DATA_BLOCK DB 20
NAME : DB_LED
VERSION : 0.1


  STRUCT
   LED_0_0 : BOOL ;
   LED_0_1 : BOOL ;
   LED_0_2 : BOOL ;
   LED_0_3 : BOOL ;
   LED_0_4 : BOOL ;
   LED_0_5 : BOOL ;
   LED_0_6 : BOOL ;
   LED_0_7 : BOOL ;
   LED_1_0 : BOOL ;
   LED_1_1 : BOOL ;
   LED_1_2 : BOOL ;
   LED_1_3 : BOOL ;
   LED_1_4 : BOOL ;
   LED_1_5 : BOOL ;
   LED_1_6 : BOOL ;
   LED_1_7 : BOOL ;
   LED_2_0 : BOOL ;
   LED_2_1 : BOOL ;
   LED_2_2 : BOOL ;
   LED_2_3 : BOOL ;
   LED_2_4 : BOOL ;
   LED_2_5 : BOOL ;
   LED_2_6 : BOOL ;
   LED_2_7 : BOOL ;
   LED_3_0 : BOOL ;
   LED_3_1 : BOOL ;
   LED_3_2 : BOOL ;
   LED_3_3 : BOOL ;
   LED_3_4 : BOOL ;
   LED_3_5 : BOOL ;
   LED_3_6 : BOOL ;
   LED_3_7 : BOOL ;
   LED_4_0 : BOOL ;
   LED_4_1 : BOOL ;
   LED_4_2 : BOOL ;
   LED_4_3 : BOOL ;
   LED_4_4 : BOOL ;
   LED_4_5 : BOOL ;
   LED_4_6 : BOOL ;
   LED_4_7 : BOOL ;
   LED_5_0 : BOOL ;
   LED_5_1 : BOOL ;
   LED_5_2 : BOOL ;
   LED_5_3 : BOOL ;
   LED_5_4 : BOOL ;
   LED_5_5 : BOOL ;
   LED_5_6 : BOOL ;
   LED_5_7 : BOOL ;
   LED_6_0 : BOOL ;
   LED_6_1 : BOOL ;
   LED_6_2 : BOOL ;
   LED_6_3 : BOOL ;
   LED_6_4 : BOOL ;
   LED_6_5 : BOOL ;
   LED_6_6 : BOOL ;
   LED_6_7 : BOOL ;
   LED_7_0 : BOOL ;
   LED_7_1 : BOOL ;
   LED_7_2 : BOOL ;
   LED_7_3 : BOOL ;
   LED_7_4 : BOOL ;
   LED_7_5 : BOOL ;
   LED_7_6 : BOOL ;
   LED_7_7 : BOOL ;
   LED_8_0 : BOOL ;
   LED_8_1 : BOOL ;
   LED_8_2 : BOOL ;
   LED_8_3 : BOOL ;
   LED_8_4 : BOOL ;
   LED_8_5 : BOOL ;
   LED_8_6 : BOOL ;
   LED_8_7 : BOOL ;
   LED_9_0 : BOOL ;
   LED_9_1 : BOOL ;
   LED_9_2 : BOOL ;
   LED_9_3 : BOOL ;
   LED_9_4 : BOOL ;
   LED_9_5 : BOOL ;
   LED_9_6 : BOOL ;
   LED_9_7 : BOOL ;
   LED_10_0 : BOOL ;
   LED_10_1 : BOOL ;
   LED_10_2 : BOOL ;
   LED_10_3 : BOOL ;
   LED_10_4 : BOOL ;
   LED_10_5 : BOOL ;
   LED_10_6 : BOOL ;
   LED_10_7 : BOOL ;
   LED_11_0 : BOOL ;
   LED_11_1 : BOOL ;
   LED_11_2 : BOOL ;
   LED_11_3 : BOOL ;
   LED_11_4 : BOOL ;
   LED_11_5 : BOOL ;
   LED_11_6 : BOOL ;
   LED_11_7 : BOOL ;
   LED_12_0 : BOOL ;
   LED_12_1 : BOOL ;
   LED_12_2 : BOOL ;
   LED_12_3 : BOOL ;
   LED_12_4 : BOOL ;
   LED_12_5 : BOOL ;
   LED_12_6 : BOOL ;
   LED_12_7 : BOOL ;
   LED_13_0 : BOOL ;
   LED_13_1 : BOOL ;
   LED_13_2 : BOOL ;
   LED_13_3 : BOOL ;
   LED_13_4 : BOOL ;
   LED_13_5 : BOOL ;
   LED_13_6 : BOOL ;
   LED_13_7 : BOOL ;
   LED_14_0 : BOOL ;
   LED_14_1 : BOOL ;
   LED_14_2 : BOOL ;
   LED_14_3 : BOOL ;
   LED_14_4 : BOOL ;
   LED_14_5 : BOOL ;
   LED_14_6 : BOOL ;
   LED_14_7 : BOOL ;
   LED_15_0 : BOOL ;
   LED_15_1 : BOOL ;
   LED_15_2 : BOOL ;
   LED_15_3 : BOOL ;
   LED_15_4 : BOOL ;
   LED_15_5 : BOOL ;
   LED_15_6 : BOOL ;
   LED_15_7 : BOOL ;
   LED_16_0 : BOOL ;
   LED_16_1 : BOOL ;
   LED_16_2 : BOOL ;
   LED_16_3 : BOOL ;
   LED_16_4 : BOOL ;
   LED_16_5 : BOOL ;
   LED_16_6 : BOOL ;
   LED_16_7 : BOOL ;
   LED_17_0 : BOOL ;
   LED_17_1 : BOOL ;
   LED_17_2 : BOOL ;
   LED_17_3 : BOOL ;
   LED_17_4 : BOOL ;
   LED_17_5 : BOOL ;
   LED_17_6 : BOOL ;
   LED_17_7 : BOOL ;
   LED_18_0 : BOOL ;
   LED_18_1 : BOOL ;
   LED_18_2 : BOOL ;
   LED_18_3 : BOOL ;
   LED_18_4 : BOOL ;
   LED_18_5 : BOOL ;
   LED_18_6 : BOOL ;
   LED_18_7 : BOOL ;
   LED_19_0 : BOOL ;
   LED_19_1 : BOOL ;
   LED_19_2 : BOOL ;
   LED_19_3 : BOOL ;
   LED_19_4 : BOOL ;
   LED_19_5 : BOOL ;
   LED_19_6 : BOOL ;
   LED_19_7 : BOOL ;
   LED_20_0 : BOOL ;
   LED_20_1 : BOOL ;
   LED_20_2 : BOOL ;
   LED_20_3 : BOOL ;
   LED_20_4 : BOOL ;
   LED_20_5 : BOOL ;
   LED_20_6 : BOOL ;
   LED_20_7 : BOOL ;
   LED_21_0 : BOOL ;
   LED_21_1 : BOOL ;
   LED_21_2 : BOOL ;
   LED_21_3 : BOOL ;
   LED_21_4 : BOOL ;
   LED_21_5 : BOOL ;
   LED_21_6 : BOOL ;
   LED_21_7 : BOOL ;
  END_STRUCT ;
BEGIN
   LED_0_0 := FALSE;
   LED_0_1 := FALSE;
   LED_0_2 := FALSE;
   LED_0_3 := FALSE;
   LED_0_4 := FALSE;
   LED_0_5 := FALSE;
   LED_0_6 := FALSE;
   LED_0_7 := FALSE;
   LED_1_0 := FALSE;
   LED_1_1 := FALSE;
   LED_1_2 := FALSE;
   LED_1_3 := FALSE;
   LED_1_4 := FALSE;
   LED_1_5 := FALSE;
   LED_1_6 := FALSE;
   LED_1_7 := FALSE;
   LED_2_0 := FALSE;
   LED_2_1 := FALSE;
   LED_2_2 := FALSE;
   LED_2_3 := FALSE;
   LED_2_4 := FALSE;
   LED_2_5 := FALSE;
   LED_2_6 := FALSE;
   LED_2_7 := FALSE;
   LED_3_0 := FALSE;
   LED_3_1 := FALSE;
   LED_3_2 := FALSE;
   LED_3_3 := FALSE;
   LED_3_4 := FALSE;
   LED_3_5 := FALSE;
   LED_3_6 := FALSE;
   LED_3_7 := FALSE;
   LED_4_0 := FALSE;
   LED_4_1 := FALSE;
   LED_4_2 := FALSE;
   LED_4_3 := FALSE;
   LED_4_4 := FALSE;
   LED_4_5 := FALSE;
   LED_4_6 := FALSE;
   LED_4_7 := FALSE;
   LED_5_0 := FALSE;
   LED_5_1 := FALSE;
   LED_5_2 := FALSE;
   LED_5_3 := FALSE;
   LED_5_4 := FALSE;
   LED_5_5 := FALSE;
   LED_5_6 := FALSE;
   LED_5_7 := FALSE;
   LED_6_0 := FALSE;
   LED_6_1 := FALSE;
   LED_6_2 := FALSE;
   LED_6_3 := FALSE;
   LED_6_4 := FALSE;
   LED_6_5 := FALSE;
   LED_6_6 := FALSE;
   LED_6_7 := FALSE;
   LED_7_0 := FALSE;
   LED_7_1 := FALSE;
   LED_7_2 := FALSE;
   LED_7_3 := FALSE;
   LED_7_4 := FALSE;
   LED_7_5 := FALSE;
   LED_7_6 := FALSE;
   LED_7_7 := FALSE;
   LED_8_0 := FALSE;
   LED_8_1 := FALSE;
   LED_8_2 := FALSE;
   LED_8_3 := FALSE;
   LED_8_4 := FALSE;
   LED_8_5 := FALSE;
   LED_8_6 := FALSE;
   LED_8_7 := FALSE;
   LED_9_0 := FALSE;
   LED_9_1 := FALSE;
   LED_9_2 := FALSE;
   LED_9_3 := FALSE;
   LED_9_4 := FALSE;
   LED_9_5 := FALSE;
   LED_9_6 := FALSE;
   LED_9_7 := FALSE;
   LED_10_0 := FALSE;
   LED_10_1 := FALSE;
   LED_10_2 := FALSE;
   LED_10_3 := FALSE;
   LED_10_4 := FALSE;
   LED_10_5 := FALSE;
   LED_10_6 := FALSE;
   LED_10_7 := FALSE;
   LED_11_0 := FALSE;
   LED_11_1 := FALSE;
   LED_11_2 := FALSE;
   LED_11_3 := FALSE;
   LED_11_4 := FALSE;
   LED_11_5 := FALSE;
   LED_11_6 := FALSE;
   LED_11_7 := FALSE;
   LED_12_0 := FALSE;
   LED_12_1 := FALSE;
   LED_12_2 := FALSE;
   LED_12_3 := FALSE;
   LED_12_4 := FALSE;
   LED_12_5 := FALSE;
   LED_12_6 := FALSE;
   LED_12_7 := FALSE;
   LED_13_0 := FALSE;
   LED_13_1 := FALSE;
   LED_13_2 := FALSE;
   LED_13_3 := FALSE;
   LED_13_4 := FALSE;
   LED_13_5 := FALSE;
   LED_13_6 := FALSE;
   LED_13_7 := FALSE;
   LED_14_0 := FALSE;
   LED_14_1 := FALSE;
   LED_14_2 := FALSE;
   LED_14_3 := FALSE;
   LED_14_4 := FALSE;
   LED_14_5 := FALSE;
   LED_14_6 := FALSE;
   LED_14_7 := FALSE;
   LED_15_0 := FALSE;
   LED_15_1 := FALSE;
   LED_15_2 := FALSE;
   LED_15_3 := FALSE;
   LED_15_4 := FALSE;
   LED_15_5 := FALSE;
   LED_15_6 := FALSE;
   LED_15_7 := FALSE;
   LED_16_0 := FALSE;
   LED_16_1 := FALSE;
   LED_16_2 := FALSE;
   LED_16_3 := FALSE;
   LED_16_4 := FALSE;
   LED_16_5 := FALSE;
   LED_16_6 := FALSE;
   LED_16_7 := FALSE;
   LED_17_0 := FALSE;
   LED_17_1 := FALSE;
   LED_17_2 := FALSE;
   LED_17_3 := FALSE;
   LED_17_4 := FALSE;
   LED_17_5 := FALSE;
   LED_17_6 := FALSE;
   LED_17_7 := FALSE;
   LED_18_0 := FALSE;
   LED_18_1 := FALSE;
   LED_18_2 := FALSE;
   LED_18_3 := FALSE;
   LED_18_4 := FALSE;
   LED_18_5 := FALSE;
   LED_18_6 := FALSE;
   LED_18_7 := FALSE;
   LED_19_0 := FALSE;
   LED_19_1 := FALSE;
   LED_19_2 := FALSE;
   LED_19_3 := FALSE;
   LED_19_4 := FALSE;
   LED_19_5 := FALSE;
   LED_19_6 := FALSE;
   LED_19_7 := FALSE;
   LED_20_0 := FALSE;
   LED_20_1 := FALSE;
   LED_20_2 := FALSE;
   LED_20_3 := FALSE;
   LED_20_4 := FALSE;
   LED_20_5 := FALSE;
   LED_20_6 := FALSE;
   LED_20_7 := FALSE;
   LED_21_0 := FALSE;
   LED_21_1 := FALSE;
   LED_21_2 := FALSE;
   LED_21_3 := FALSE;
   LED_21_4 := FALSE;
   LED_21_5 := FALSE;
   LED_21_6 := FALSE;
   LED_21_7 := FALSE;
END_DATA_BLOCK

